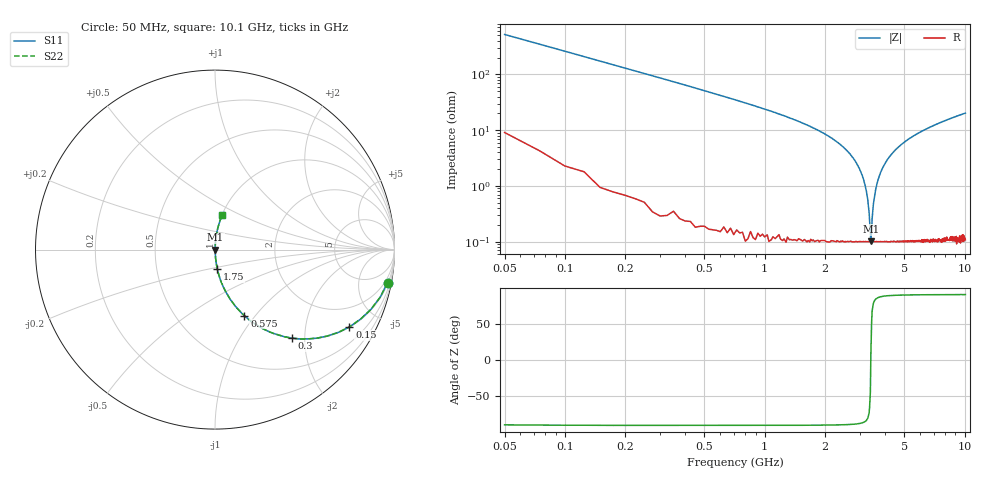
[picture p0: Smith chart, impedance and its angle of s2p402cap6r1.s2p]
! AVX Thin Film Operation		Date: April 2003
! Description: Accu-P® Series, Thin Film, SMD, RF Capacitor
! Part Number: 0402ZK6R1BBW
! 50 MHz  -  10.05 GHz
! Serial Measurements
# hz S db R 50
!	S11		S21		S12		S22
!	dB	Phase	dB	Phase	dB	Phase	dB	Phase
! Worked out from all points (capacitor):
!   400 points, 50 MHz to 10.1 GHz, reference 50 ohm
!   read as one part in series: C = 6.1 pF near 100 MHz
!   lowest |Z| = 101 mohm at 3.4 GHz (marker M1)
!   series resonance near 3.397 GHz, so ESL is about 360 pH
!   S11 on the Smith chart (normalised r, x): 50 MHz: 1, -10; 150 MHz: 1.02, -3.47; 300 MHz: 1.01, -1.73; 575 MHz: 1.00, -0.88; 1.75 GHz: 1.00, -0.22; 10.1 GHz: 1.00, +0.40
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5e7  -0.18 -10.8  -14.50 78.2  -14.50 78.2  -0.18 -10.8
1e8  -0.62 -20.9  -8.94 68.6  -8.94 68.6  -0.62 -20.9
1.5e8  -1.27 -29.9  -6.06 59.8  -6.06 59.8  -1.27 -29.9
3e8  -3.71 -49.1  -2.43 40.7  -2.43 40.7  -3.71 -49.1
5.75e8  -7.90 -66.0  -0.78 23.8  -0.78 23.8  -7.90 -66.0
9.75e8  -12.50 -75.9  -0.26 13.8  -0.26 13.8  -12.50 -75.9
1.73e9  -19.10 -83.1  -0.06 6.4  -0.06 6.4  -19.10 -83.1
1.75e9  -19.30 -83.2  -0.06 6.2  -0.06 6.2  -19.30 -83.2
2.58e9  -27.30 -86.2  -0.02 2.5  -0.02 2.5  -27.30 -86.2
3.03e9  -35.00 -85.8  -0.01 1.0  -0.01 1.0  -35.00 -85.8
3.18e9  -39.70 -83.9  -0.01 0.6  -0.01 0.6  -39.70 -83.9
3.28e9  -44.90 -79.5  -0.01 0.3  -0.01 0.3  -44.90 -79.5
3.33e9  -49.40 -72.8  -0.01 0.2  -0.01 0.2  -49.40 -72.8
3.4e9  -59.90 9.5  -0.01 -0.0  -0.01 -0.0  -59.90 9.5
3.45e9  -51.70 67.3  -0.01 -0.1  -0.01 -0.1  -51.70 67.3
3.55e9  -43.30 81.2  -0.01 -0.4  -0.01 -0.4  -43.30 81.2
3.8e9  -35.20 85.7  -0.01 -1.0  -0.01 -1.0  -35.20 85.7
4.3e9  -28.70 86.3  -0.01 -2.1  -0.01 -2.1  -28.70 86.3
5.08e9  -24.00 85.5  -0.03 -3.6  -0.03 -3.6  -24.00 85.5
6.75e9  -18.90 83.0  -0.07 -6.5  -0.07 -6.5  -18.90 83.0
8.43e9  -16.10 80.6  -0.12 -9.1  -0.12 -9.1  -16.10 80.6
1.01e10  -14.10 78.3  -0.18 -11.4  -0.18 -11.4  -14.10 78.3
